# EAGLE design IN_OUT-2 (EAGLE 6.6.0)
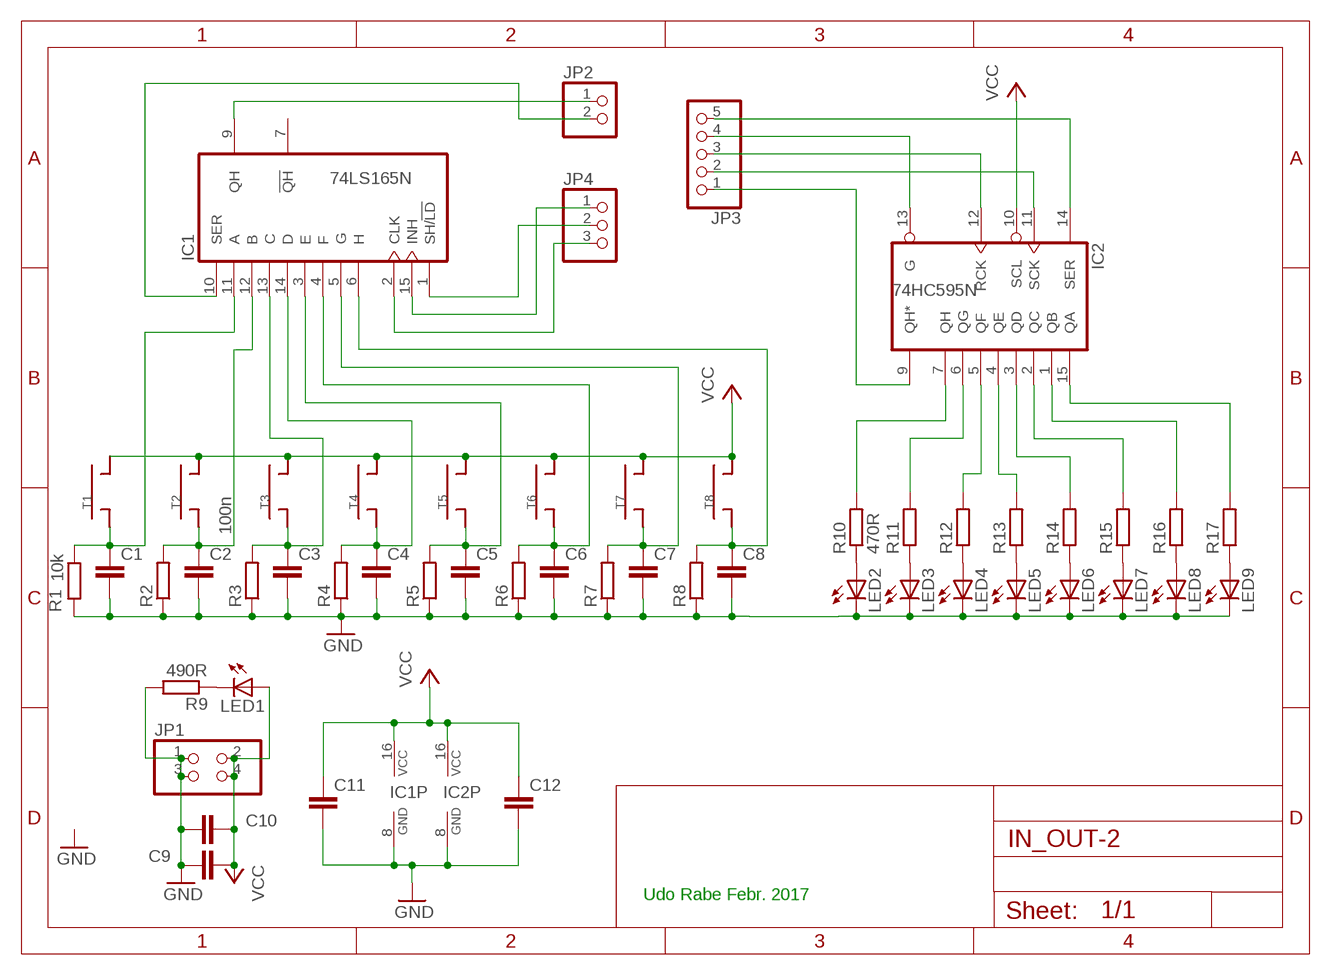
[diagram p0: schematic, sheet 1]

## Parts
C1  C-EU075-032X103  [C075-032X103]
C2  100n  C-EU075-032X103  [C075-032X103]
C3  C-EU075-032X103  [C075-032X103]
C4  C-EU075-032X103  [C075-032X103]
C5  C-EU075-032X103  [C075-032X103]
C6  C-EU075-032X103  [C075-032X103]
C7  C-EU075-032X103  [C075-032X103]
C8  C-EU075-032X103  [C075-032X103]
C9  C-EU025-025X050  [C025-025X050]
C10  C-EU025-025X050  [C025-025X050]
C11  C-EU075-032X103  [C075-032X103]
C12  C-EU075-032X103  [C075-032X103]
IC1  74LS165N  [DIL16]
IC2  74HC595N  [DIL16]
JP1  PINHD-2X2  [2X02]
JP2  PINHD-1X2  [1X02]
JP3  PINHD-1X5  [1X05]
JP4  PINHD-1X3  [1X03]
LED1  LED3MM  [LED3MM]
LED2  LED5MM  [LED5MM]
LED3  LED5MM  [LED5MM]
LED4  LED5MM  [LED5MM]
LED5  LED5MM  [LED5MM]
LED6  LED5MM  [LED5MM]
LED7  LED5MM  [LED5MM]
LED8  LED5MM  [LED5MM]
LED9  LED5MM  [LED5MM]
R1  10k  R-EU_0207/10  [0207/10]
R2  R-EU_0207/10  [0207/10]
R3  R-EU_0207/10  [0207/10]
R4  R-EU_0207/10  [0207/10]
R5  R-EU_0207/10  [0207/10]
R6  R-EU_0207/10  [0207/10]
R7  R-EU_0207/10  [0207/10]
R8  R-EU_0207/10  [0207/10]
R9  490R  R-EU_0207/10  [0207/10]
R10  470R  R-EU_0207/10  [0207/10]
R11  R-EU_0207/10  [0207/10]
R12  R-EU_0207/10  [0207/10]
R13  R-EU_0207/10  [0207/10]
R14  R-EU_0207/10  [0207/10]
R15  R-EU_0207/10  [0207/10]
R16  R-EU_0207/10  [0207/10]
R17  R-EU_0207/10  [0207/10]
T1  T  [TAST90]
T2  T  [TAST90]
T3  T  [TAST90]
T4  T  [TAST90]
T5  T  [TAST90]
T6  T  [TAST90]
T7  T  [TAST90]
T8  T  [TAST90]

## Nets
GND: C1.2 C2.2 C3.2 C4.2 C5.2 C6.2 C7.2 C8.2 C9.1 C10.1 C11.2 C12.2 IC1.8(GND) IC2.8(GND) JP1.1 JP1.3 LED2.K(C) LED3.K(C) LED4.K(C) LED5.K(C) LED6.K(C) LED7.K(C) LED8.K(C) LED9.K(C) R1.2 R2.1 R3.1 R4.1 R5.1 R6.1 R7.1 R8.1 R9.2
N$1: C1.1 IC1.11(A) R1.1 T1.PIN2
N$2: C2.1 IC1.12(B) R2.2 T2.PIN2
N$3: C3.1 IC1.13(C) R3.2 T3.PIN2
N$4: C4.1 IC1.14(D) R4.2 T4.PIN2
N$5: C5.1 IC1.3(E) R5.2 T5.PIN2
N$6: C6.1 IC1.4(F) R6.2 T6.PIN2
N$7: C7.1 IC1.5(G) R7.2 T7.PIN2
N$8: C8.1 IC1.6(H) R8.2 T8.PIN2
N$9: LED2.A R10.1
N$10: IC2.13(G) JP3.4
N$11: IC2.11(SCK) JP3.2
N$18: LED9.A R17.1
N$19: LED1.K(C) R9.1
N$20: IC2.7(QH) R10.2
N$21: IC2.6(QG) R11.2
N$22: LED8.A R16.1
N$23: LED7.A R15.1
N$24: LED6.A R14.1
N$25: LED5.A R13.1
N$26: LED4.A R12.1
N$27: LED3.A R11.1
N$28: IC2.5(QF) R12.2
N$29: IC2.4(QE) R13.2
N$30: IC2.3(QD) R14.2
N$31: IC2.2(QC) R15.2
N$32: IC2.1(QB) R16.2
N$33: IC2.15(QA) R17.2
N$34: IC2.9(QH*) JP3.1
N$35: IC2.12(RCK) JP3.3
N$37: IC2.14(SER) JP3.5
N$38: IC1.10(SER) JP2.2
N$39: IC1.1(SH/!LD) JP4.2
N$40: IC1.15(INH) JP4.1
N$41: IC1.2(CLK) JP4.3
N$42: IC1.9(QH) JP2.1
VCC: C9.2 C10.2 C11.1 C12.1 IC1.16(VCC) IC2.10(SCL) IC2.16(VCC) JP1.2 JP1.4 LED1.A T1.PIN1 T2.PIN1 T3.PIN1 T4.PIN1 T5.PIN1 T6.PIN1 T7.PIN1 T8.PIN1
Unconnected: IC1.7(!QH)

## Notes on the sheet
- Udo Rabe Febr. 2017

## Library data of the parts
C1-C12 = rcl:C-EU: CAPACITOR, European symbol
IC1 = 74xx-eu:74*165: 8-bit parallel load SHIFT REGISTER
IC2 = 74xx-eu:74*595: 8-bit SHIFT REGISTER, output latch
JP1 = pinhead:PINHD-2X2: PIN HEADER
JP2 = pinhead:PINHD-1X2: PIN HEADER
JP3 = pinhead:PINHD-1X5: PIN HEADER
JP4 = pinhead:PINHD-1X3: PIN HEADER
LED1-LED9 = led:LED: LED
R1-R17 = rcl:R-EU_: RESISTOR, European symbol
T1-T8 = mylbr:T

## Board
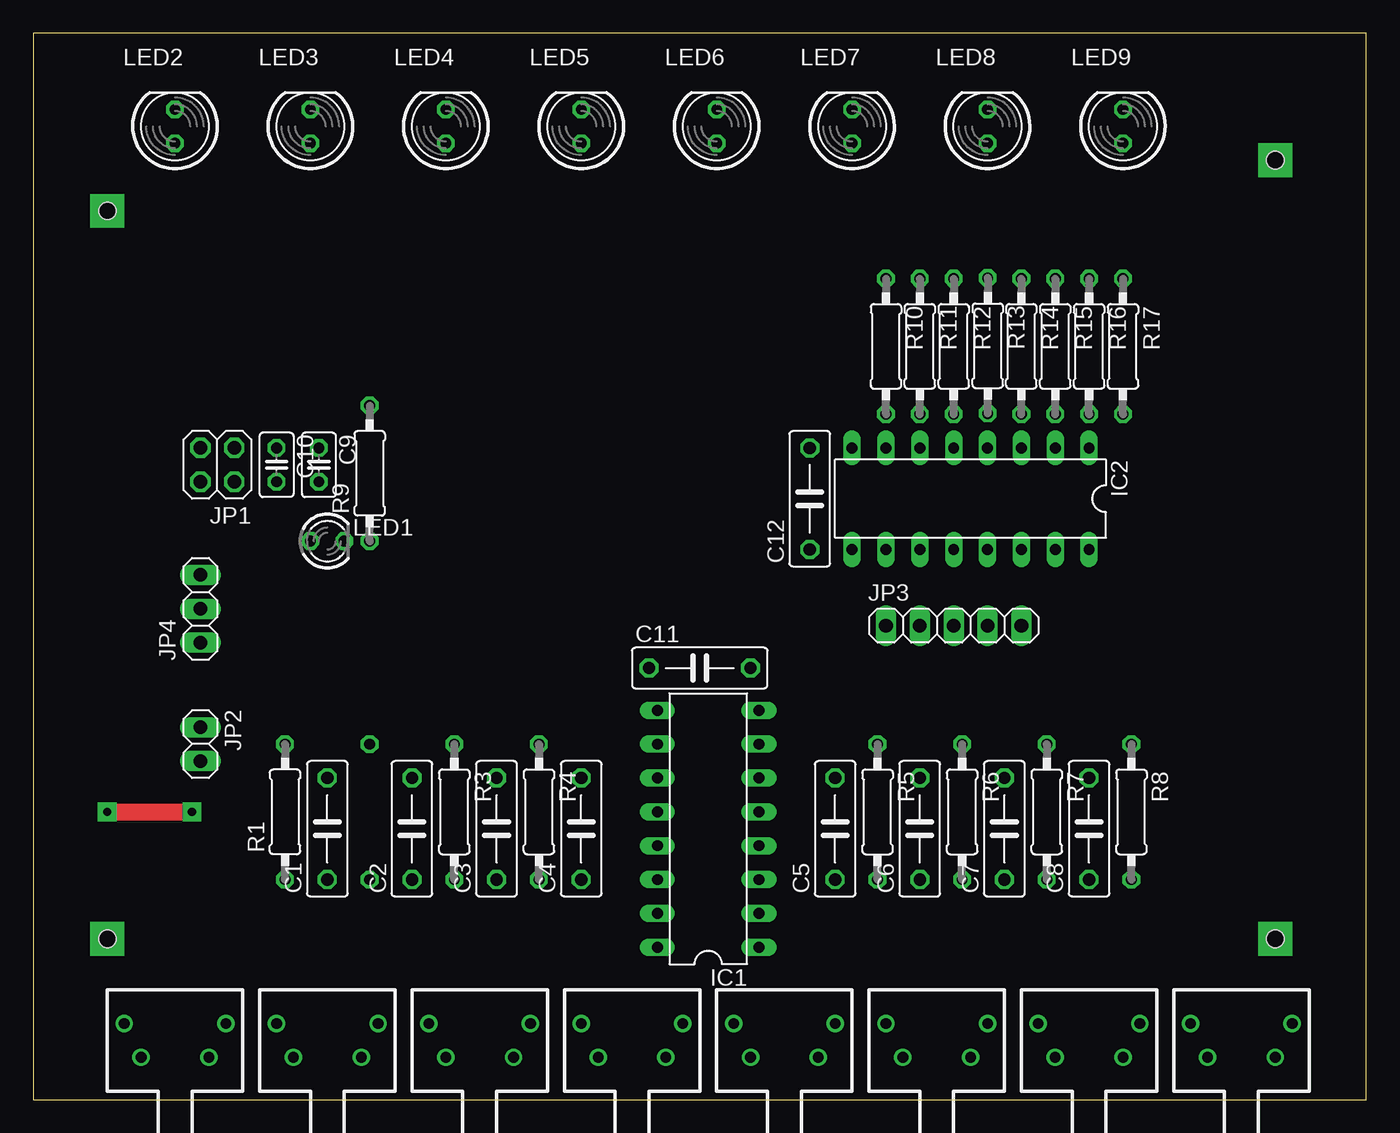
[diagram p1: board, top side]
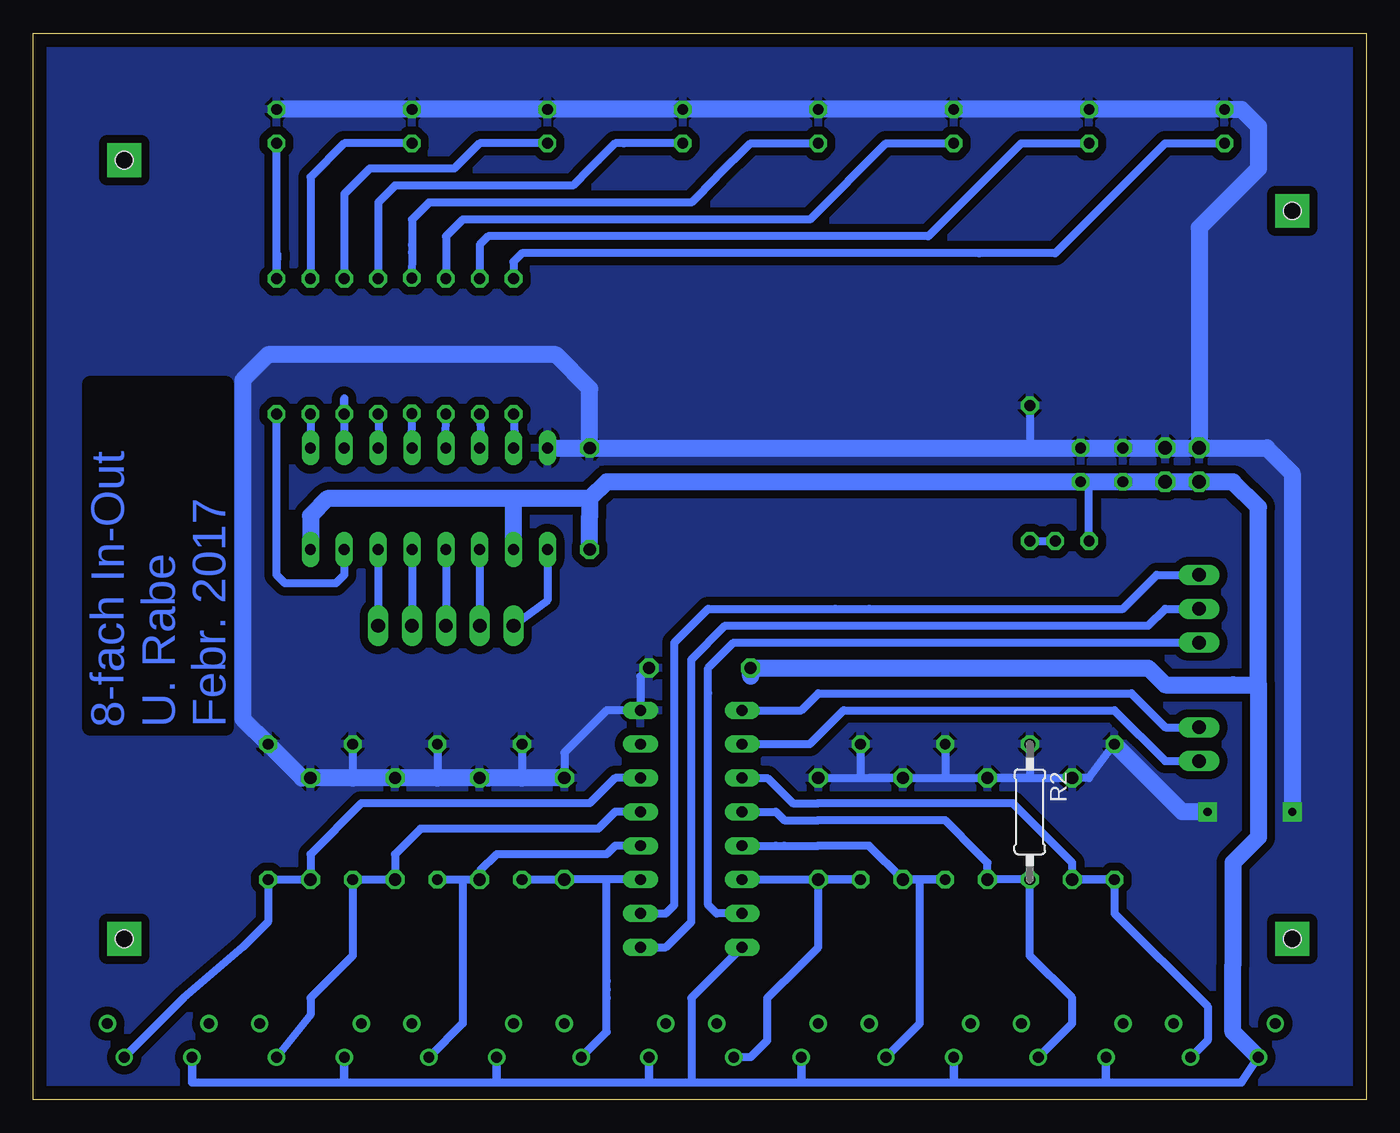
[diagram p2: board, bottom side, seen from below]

Size 100 x 80 mm. Coordinates in mm from the lower left corner, seen from the top.
Outline: 0,0 100,0 100,80 0,80 0,0
Copper layers (1*16): Top 0.035mm / dielectric 1.5mm / Bottom 0.035mm
Design rules "default *": minimum track width 24mil, minimum drill 24mil, track to track 8mil, track to pad 8mil, pad to pad 8mil, via to via 8mil, smd to smd 8mil, copper to edge 40mil, drill to drill 8mil, minimum pad ring 10mil, minimum via ring 8mil, stop-mask expansion 4mil, vias tented up to drill 0mil, thermal gap 10mil
Holes 1.3 mm at 5.55,12.06 93.18,12.06 93.18,70.48 5.55,66.67

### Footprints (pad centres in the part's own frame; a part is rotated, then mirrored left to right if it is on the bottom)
C075-032X103 = drill 0.914 octagon: 1 -3.81,0; 2 3.81,0
C025-025X050 = drill 0.813 octagon: 1 -1.27,0; 2 1.27,0
DIL16 = drill 0.813 long: 1 -8.89,-3.81; 2 -6.35,-3.81; 3 -3.81,-3.81; 4 -1.27,-3.81; 5 1.27,-3.81; 6 3.81,-3.81; 7 6.35,-3.81; 8 8.89,-3.81; 9 8.89,3.81; 10 6.35,3.81; 11 3.81,3.81; 12 1.27,3.81; 13 -1.27,3.81; 14 -3.81,3.81; 15 -6.35,3.81; 16 -8.89,3.81
2X02 = drill 1.016 octagon: 1 -1.27,-1.27; 2 -1.27,1.27; 3 1.27,-1.27; 4 1.27,1.27
1X02 = drill 1.016 long: 1 -1.27,0; 2 1.27,0
1X05 = drill 1.016 long: 1 -5.08,0; 2 -2.54,0; 3 0,0; 4 2.54,0; 5 5.08,0
1X03 = drill 1.016 long: 1 -2.54,0; 2 0,0; 3 2.54,0
LED3MM = drill 0.813 octagon: A -1.27,0; K 1.27,0
LED5MM = drill 0.813 octagon: A -1.27,0; K 1.27,0
0207/10 = drill 0.813 octagon: 1 -5.08,0; 2 5.08,0
TAST90 = drill 0.8: P3 -3.81,2.54; P4 3.81,2.54; PIN1 -2.54,0; PIN2 2.54,0

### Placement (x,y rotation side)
C1  22.06,20.32 90 top
C2  28.41,20.32 90 top
C3  34.76,20.32 90 top
C4  41.11,20.32 90 top
C5  60.16,20.32 90 top
C6  66.51,20.32 90 top
C7  72.86,20.32 90 top
C8  79.21,20.32 90 top
C9  21.43,47.62 270 top
C10  18.25,47.62 270 top
C11  50,32.38 0 top
C12  58.26,45.08 90 top
IC1  50.63,20.32 90 top
IC2  70.32,45.08 180 top
JP1  13.81,47.62 180 top
JP2  12.54,26.67 270 top
JP3  69.05,35.55 0 top
JP4  12.54,36.82 90 top
LED1  22.06,41.9 0 top
LED2  10.63,73.02 90 top
LED3  20.79,73.02 90 top
LED4  30.95,73.02 90 top
LED5  41.11,73.02 90 top
LED6  51.27,73.02 90 top
LED7  61.43,73.02 90 top
LED8  71.59,73.02 90 top
LED9  81.75,73.02 90 top
R1  18.89,21.59 90 top
R2  25.23,21.59 270 bottom
R3  31.59,21.59 270 top
R4  37.94,21.59 270 top
R5  63.34,21.59 270 top
R6  69.68,21.59 270 top
R7  76.03,21.59 270 top
R8  82.38,21.59 270 top
R9  25.23,46.98 90 top
R10  63.97,56.51 270 top
R11  66.51,56.51 270 top
R12  69.05,56.51 270 top
R13  71.6,56.56 270 top
R14  74.13,56.51 270 top
R15  76.67,56.51 270 top
R16  79.21,56.51 270 top
R17  81.75,56.51 270 top
T1  10.63,3.17 0 top
T2  22.06,3.17 0 top
T3  33.49,3.17 0 top
T4  44.92,3.17 0 top
T5  56.35,3.17 0 top
T6  67.78,3.17 0 top
T7  79.21,3.17 0 top
T8  90.64,3.17 0 top

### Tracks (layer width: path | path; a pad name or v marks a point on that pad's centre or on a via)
GND  (via drill 0.61 pad 1.42)
  Top 1.27: v5.55,21.59 v11.9,21.59
  Bottom 0.61: C4.2 37.94,24.12 | 37.94,24.12 37.3,24.12 | 37.3,24.12 C3.2 | C3.2 31.59,24.12 | 31.59,24.12 C2.2 | C2.2 C1.2 20.79,24.12 R1.2 | R2.1 25.23,24.12 C2.2 | R3.1 31.59,24.12 | R4.1 37.94,24.12 | 79.84,24.12 C8.2 | R7.1 76.03,24.12 | R6.1 69.68,24.12 C7.2 | R5.1 63.34,24.12 65.88,24.12 C6.2 | C5.2 60.16,26.03 56.98,29.21 IC1.8 54.45,31.75 C11.2 | R9.2 25.23,48.89 | C3.2 37.3,24.12
  Bottom 1.27: LED9.K LED8.K LED7.K LED6.K LED5.K LED4.K LED3.K LED2.K 9.36,74.29 8.09,73.02 8.09,69.84 12.54,65.4 JP1.3 | IC2.8 C12.2 | C5.2 63.34,24.12 65.88,24.12 C6.2 69.68,24.12 C7.2 76.03,24.12 C8.2 | 79.84,24.12 R8.1 84.29,28.57 84.29,53.97 82.38,55.88 60.8,55.88 58.26,53.34 C12.2 | C12.2 25.23,48.89 C9.1 C10.1 JP1.1 JP1.3 | 11.9,48.89 JP1.3 | JP1.3 7.46,48.89 5.55,46.98 v5.55,21.59 | v11.9,21.59 13.81,21.59 R1.2
  pour Bottom (isolate 0.61): -0.8,80.64 101.43,80.64 101.43,-0.64 -0.8,-0.64
N$1
  Bottom 0.61: 12.54,3.81 T1.PIN2 11.9,4.44 11.9,6.98 18.89,13.96 18.89,15.87 R1.1 | R1.1 C1.1 | C1.1 R1.1 | R1.1 C1.1 | C1.1 22.06,17.78 26.51,22.22 41.11,22.22 43.02,22.22 44.92,24.12 IC1.11
N$2
  Bottom 0.61: T2.PIN2 22.06,5.71 22.06,7.62 25.23,10.79 R2.2 C2.1 28.41,17.78 29.05,18.41 31.59,20.95 34.12,20.95 41.11,20.95 43.65,20.95 44.29,21.59 IC1.12
N$3
  Bottom 0.61: T3.PIN2 33.49,5.71 33.49,7.62 33.49,8.25 33.49,9.52 33.49,16.51 | 33.49,16.51 R3.2 33.49,16.51 | 33.49,16.51 C3.1 | 33.49,16.51 C3.1 | C3.1 33.49,16.51 | C3.1 37.3,19.05 37.94,19.05 41.11,19.05 43.65,19.05 44.29,19.05 IC1.13
N$4
  Bottom 0.61: T4.PIN2 46.19,3.17 44.92,4.44 44.92,5.08 44.92,7.62 42.38,10.15 41.11,11.42 C4.1 | R4.2 39.2,16.51 | 39.2,16.51 C4.1 | C4.1 R4.2 | R4.2 39.2,16.51 | IC1.14 C4.1
N$5
  Bottom 0.61: T5.PIN2 56.98,5.08 56.98,7.62 56.98,8.25 56.98,8.88 56.98,16.51 | IC1.3 56.98,16.51 | 56.98,16.51 C5.1 R5.2
N$6
  Bottom 0.61: T6.PIN2 67.78,5.71 67.78,16.51 R6.2 C6.1 66.51,17.14 65.24,18.41 56.98,18.41 56.35,19.05 IC1.4
N$7
  Bottom 0.61: T7.PIN2 79.21,6.34 79.21,7.62 76.03,10.79 R7.2 C7.1 72.86,18.41 70.95,20.32 57.62,20.32 56.35,21.59 IC1.5
N$8
  Bottom 0.61: T8.PIN2 88.73,7.62 84.29,11.42 82.38,13.33 R8.2 C8.1 79.21,18.41 75.4,22.22 58.26,22.22 56.35,24.12 IC1.6
N$9
  Bottom 0.61: LED2.A 15.08,71.75 16.98,69.84 23.33,63.49 29.05,63.49 63.34,63.49 63.97,62.86 R10.1
N$10
  Bottom 0.61: IC2.13 JP3.4
N$11
  Bottom 0.61: IC2.11 JP3.2
N$15  (via drill 1.3 pad 2.54)
  other vias: 5.55,66.67
N$16  (via drill 1.3 pad 2.54)
  other vias: 5.55,12.06
N$17  (via drill 1.3 pad 2.54)
  other vias: 93.18,12.06
N$18
  Bottom 0.61: 81.67,63.42 R17.1 LED9.A
N$19
  Bottom 0.61: R9.1 LED1.K
N$20
  Bottom 0.61: R10.2 63.86,49 IC2.7
N$21
  Bottom 0.61: R11.2 66.37,49.03 IC2.6
N$22
  Bottom 0.61: LED8.A 76.67,71.75 79.21,69.21 R16.1
N$23
  Bottom 0.61: LED7.A 66.51,71.75 68.41,69.84 74.77,69.84 76.67,67.94 R15.1
N$24
  Bottom 0.61: LED6.A 55.72,71.75 56.35,71.75 57.62,70.48 58.26,69.84 59.52,68.58 72.86,68.58 74.13,67.31 R14.1
N$25
  Bottom 0.61: LED5.A 46.19,71.75 48.74,69.23 48.74,69.2 50.63,67.31 70.32,67.31 71.59,66.04 71.59,64.13 71.59,63.56 R13.1
N$26
  Bottom 0.61: LED4.A 36.03,71.75 41.74,66.04 67.78,66.04 69.05,64.77 R12.1
N$27
  Bottom 0.61: LED3.A 25.87,71.75 29.05,68.58 32.86,64.77 65.88,64.77 66.51,64.13 R11.1
N$28
  Bottom 0.61: R12.2 69.13,49.48 IC2.5
N$29
  Bottom 0.61: R13.2 71.64,48.94 IC2.4
N$30
  Bottom 0.61: R14.2 74.02,49 IC2.3
N$31
  Bottom 0.61: IC2.2 76.67,52.6 R15.2
N$32
  Bottom 0.61: IC2.1 79.21,50.06 R16.2
N$33
  Bottom 0.61: R17.2 81.75,39.36 81.11,38.73 77.3,38.73 76.67,39.36 76.67,40 IC2.15
N$34
  Bottom 0.61: JP3.1 61.43,37.46 IC2.9
N$35
  Bottom 0.61: IC2.12 JP3.3
N$36  (via drill 1.3 pad 2.54)
  other vias: 93.18,70.48
N$37
  Bottom 0.61: IC2.14 JP3.5
N$38
  Bottom 0.61: IC1.10 41.74,26.67 39.2,29.21 18.89,29.21 15.08,25.39 JP2.2
N$39
  Bottom 0.61: IC1.1 52.54,11.42 50.63,13.33 50.63,31.11 50.63,33.02 48.09,35.55 39.2,35.55 37.3,35.55 16.35,35.55 15.08,36.82 JP4.2
N$40
  Bottom 0.61: IC1.15 48.73,13.96 49.37,14.6 49.37,30.48 49.37,32.38 47.46,34.28 37.94,34.28 36.66,34.28 22.7,34.28 18.25,34.28 JP4.1
N$41
  Bottom 0.61: IC1.2 52.54,13.96 51.91,14.6 51.91,31.11 51.91,34.28 49.37,36.82 39.84,36.82 37.3,36.82 18.25,36.82 15.71,39.36 JP4.3
N$42
  Bottom 0.61: IC1.9 42.38,29.21 41.11,30.48 17.62,30.48 15.08,27.94 JP2.1
VCC
  Bottom 0.61: 63.97,42.54 IC2.10 | 88.1,1.27 T8.PIN1 88.1,1.27 | 76.67,1.27 88.1,1.27 | 76.67,1.27 T7.PIN1 76.67,1.27 | 65.24,1.27 76.67,1.27 | 65.24,1.27 T6.PIN1 65.24,1.27 | 53.81,1.27 65.24,1.27 | 53.81,1.27 T5.PIN1 53.81,1.27 | 42.38,1.27 50,1.27 50.63,1.27 | 50.63,1.27 53.81,1.27 | 42.38,1.27 T4.PIN1 42.38,1.27 | 30.95,1.27 42.38,1.27 | 30.95,1.27 T3.PIN1 30.95,1.27 | 19.52,1.27 30.95,1.27 | 19.52,1.27 T2.PIN1 19.52,1.27 | 19.52,1.27 9.36,1.27 T1.PIN1 | IC1.16 50.63,7.62 50.63,1.27 | 58.26,43.81 58.26,45.08 | LED1.A 20.79,46.35 C10.2
  Bottom 1.27: IC2.16 79.21,43.81 77.94,45.08 63.97,45.08 | 63.97,45.08 63.97,43.81 IC2.10 | C12.1 58.26,43.81 58.26,45.08 | 58.26,45.08 63.97,45.08 | 58.26,45.08 56.98,46.35 C9.2 C10.2 JP1.2 JP1.4 10,46.35 8.09,44.45 8.09,31.11 | T1.PIN1 10,5.08 10,10.15 10,17.78 9.36,18.41 8.09,19.68 8.09,31.11 | 46.19,31.75 C11.1 16.35,32.38 15.08,31.11 10,31.11 8.09,31.11

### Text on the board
Bottom: 1 | 1 | GND | VCC | 8-fach In-Out / U. Rabe / Febr. 2017 | G | Ser | Ser | QH | RCK | SCK | QH*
